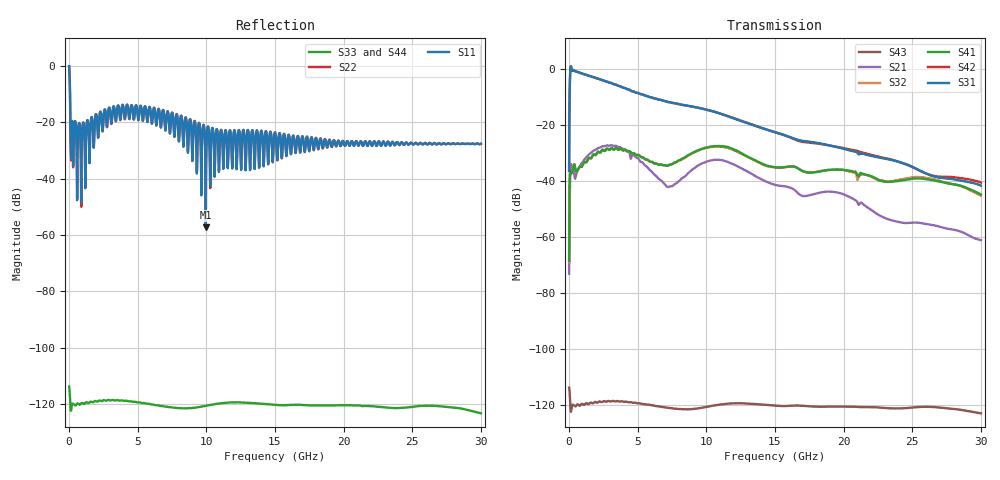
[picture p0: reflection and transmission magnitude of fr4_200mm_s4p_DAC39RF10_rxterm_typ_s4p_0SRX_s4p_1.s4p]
! Touchstone generated by fitter/viewer
# HZ S  RI R 5.000000e+01
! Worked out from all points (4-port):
!   3599 points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, 8.336 MHz to 30 GHz, reference 50 ohm
!   strongest paths, dB at 8.336 MHz, 7.502 GHz, 15 GHz, 22.51 GHz, 30 GHz:
!     S31: -36.5, -12.2, -22.7, -31.6, -41.7
!     S42: -36.5, -12.2, -22.7, -31.4, -40.6
!     S41: -68.7, -34.1, -35.2, -39.6, -44.9
!     S32: -69.1, -34.1, -35.3, -39.7, -45.3
!     S21: -73.1, -41.9, -41.5, -52.1, -61.2
!     S43: -113.8, -121.2, -120.2, -120.9, -123.0
!   lowest |S11| = -57.3 dB at 9.961 GHz (marker M1), VSWR 1.00, Z = 49.9 - j0.00172 ohm
!   |S11| at or under -10 dB: 75.14 MHz to end of sweep
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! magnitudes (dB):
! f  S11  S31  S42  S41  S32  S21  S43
! 8.336 MHz  -0.1  -36.5  -36.5  -68.7  -69.1  -73.1  -113.8
! 225.1 MHz  -19.8  -0.8  -0.7  -36.9  -36.8  -37.1  -120.1
! 2.067 GHz  -21.3  -3.5  -3.5  -29.8  -29.9  -28.5  -119.2
! 4.251 GHz  -13.9  -7.3  -7.3  -29.5  -29.5  -29.4  -118.9
! 7.227 GHz  -16.9  -11.9  -11.9  -34.5  -34.6  -42.2  -121.0
! 9.961 GHz  -57.3  -14.6  -14.6  -28.2  -28.3  -33.3  -120.7
! 30 GHz  -27.6  -41.7  -40.6  -44.9  -45.3  -61.2  -123.0
